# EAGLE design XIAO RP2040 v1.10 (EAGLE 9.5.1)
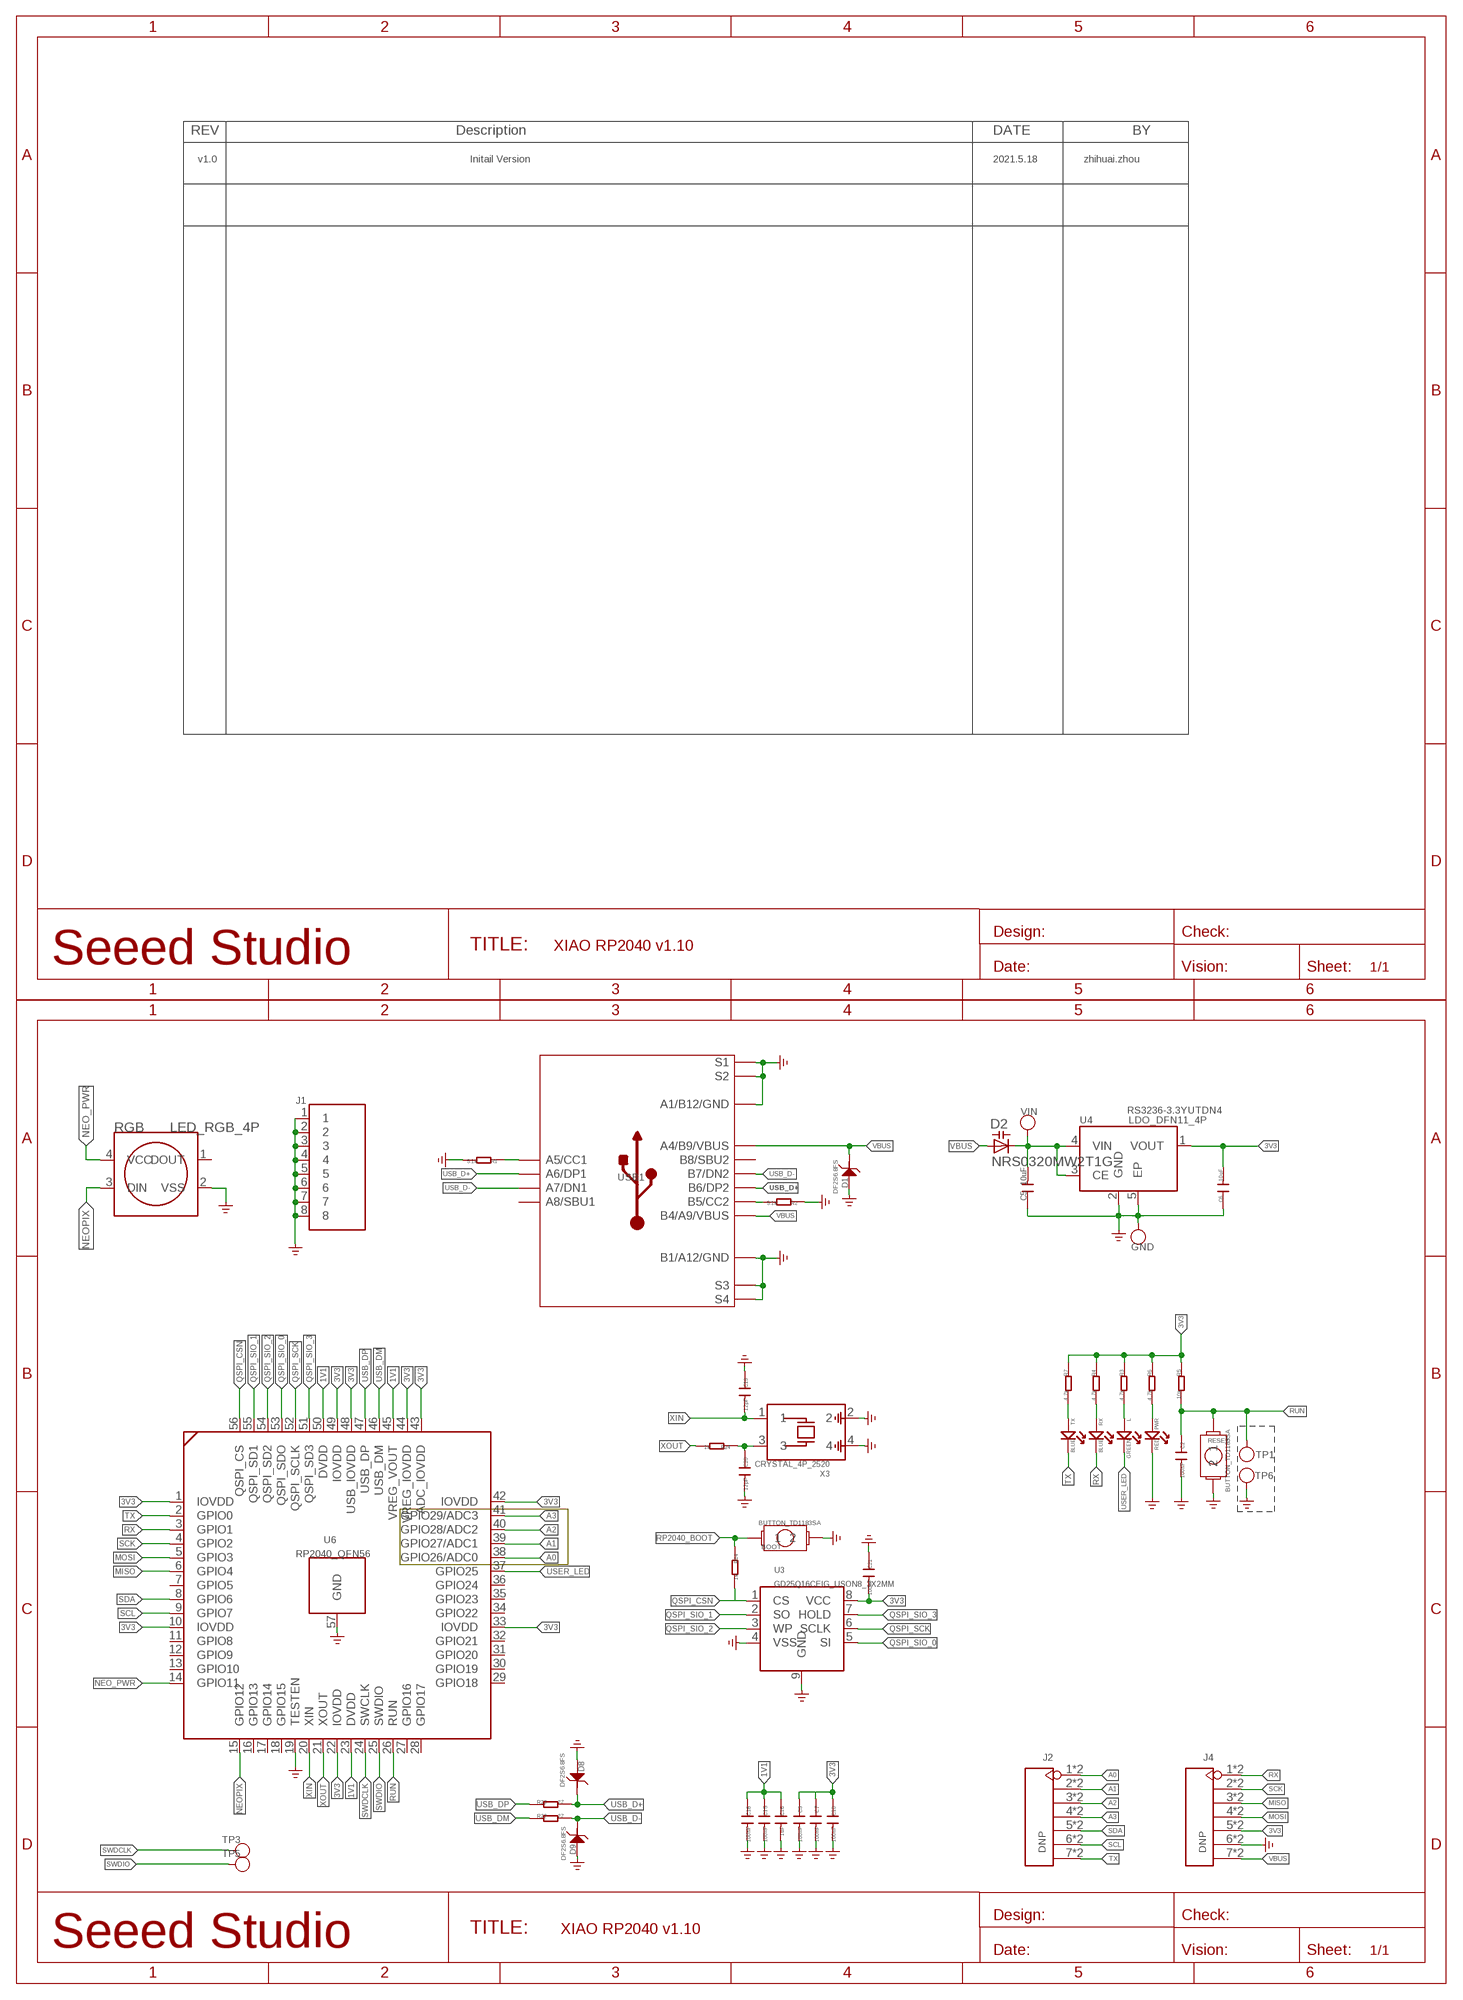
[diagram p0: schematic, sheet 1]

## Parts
BOOT  BUTTON_TD1183SA  [BUTTON_TD1183SA]
C2  100nF  CAP\0201NNS  [0201_NORMAL\NOSILK]
C3  100nF  CAP\0201NNS  [0201_NORMAL\NOSILK]
C5  10uF  C-0402  [C0402]
C6  10uF  C-0402  [C0402]
C7  100nF  CAP\0201NNS  [0201_NORMAL\NOSILK]
C10  100nF  CAP\0201NNS  [0201_NORMAL\NOSILK]
C15  100nF  CAP\0201NNS  [0201_NORMAL\NOSILK]
C16  1uF  CAP\0201NNS  [0201_NORMAL\NOSILK]
C18  100nF  CAP\0201NNS  [0201_NORMAL\NOSILK]
C19  12pF  CAP\0201NNS  [0201_NORMAL\NOSILK]
C20  12pF  CAP\0201NNS  [0201_NORMAL\NOSILK]
C21  100nF  CAP\0201NNS  [0201_NORMAL\NOSILK]
D1  DF2S6.8FS  D-ESD-2P'DF2S6.8FS'  [SOD-923]
D2  NRS0320MW2T1G  DIODE_CAPACITANCE-SOD523  [SOD523]
D8  DF2S6.8FS  D-ESD-2P'DF2S6.8FS'  [SOD-923]
D9  DF2S6.8FS  D-ESD-2P'DF2S6.8FS'  [SOD-923]
GND  TEST-POINT'4080'  [TP-80X40MIL]
J1  SHIELDING-COVER-XIAO_RP2040_PRD  [SHIELDING-COVER_XIAO_RP2040_PRD]
J2  DNP  HEADER-7P-HALF-HOLE-2.54  [H7-HALF-HOLE-2.54]
J4  DNP  HEADER-7P-HALF-HOLE-2.54  [H7-HALF-HOLE-2.54]
L  GREEN  LED-0402  [LED-0402]
PWR  RED  LED-0402  [LED-0402]
R1  5.1k  R-0201  [R0201]
R2  5.1k  R-0201  [R0201]
R3  4.7k  R-0201  [R0201]
R4  4.7k  R-0201  [R0201]
R5  10k  R-0201  [R0201]
R6  4.7k  R-0201  [R0201]
R7  4.7k  R-0201  [R0201]
R14  1k  R-0201  [R0201]
R22  27  R-0201  [R0201]
R23  27  R-0201  [R0201]
R24  1k  R-0201  [R0201]
RESET  BUTTON_TD1183SA  [BUTTON_TD1183SA]
RGB  LED_RGB_4P  [LED_RGB_2427]
RX  BLUE  LED-0402  [LED-0402]
TP1  TEST-POINT'4545'  [TP-D45MIL]
TP3  TEST-POINT'4545'  [TP-D45MIL]
TP5  TEST-POINT'4545'  [TP-D45MIL]
TP6  TEST-POINT'4545'  [TP-D45MIL]
TX  BLUE  LED-0402  [LED-0402]
U3  GD25Q16CEIG_USON8_3X2MM  [GD25Q16CEIG_USON8_3X2MM]
U4  LDO_DFN11_4P  [LDO_DFN1*1_4P]
U6  RP2040_QFN56  [RP2040_QFN56]
USB1  USB2.0-TYPE-C  [USB2.0-TYPE-C]
VIN  TEST-POINT'4080'  [TP-80X40MIL]
X3  CRYSTAL_4P_2520  [CRYSTAL_4P_2520]

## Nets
1V1: C15.1 C16.1 C18.1 U6.23(DVDD) U6.45(VREG_VOUT) U6.50(DVDD)
3V3: C3.1 C6.2 C7.1 C10.1 C21.2 J4.5 J4.17 R3.1 R4.1 R5.1 R6.1 R7.1 U3.8(VCC) U4.1(VOUT) U6.1(IOVDD) U6.10(IOVDD) U6.22(IOVDD) U6.33(IOVDD) U6.42(IOVDD) U6.43(ADC_IOVDD) U6.44(VREG_IOVDD) U6.48(USB_IOVDD) U6.49(IOVDD)
A0: J2.1 J2.13 U6.38(GPIO26/ADC0)
A1: J2.2 J2.14 U6.39(GPIO27/ADC1)
A2: J2.3 J2.15 U6.40(GPIO28/ADC2)
A3: J2.4 J2.16 U6.41(GPIO29/ADC3)
GND: BOOT.2 C2.2 C3.2 C5.1 C6.1 C7.2 C10.2 C15.2 C16.2 C18.2 C19.1 C20.2 C21.1 D1.2 D8.2 D9.2 GND.1(T) J1.1 J1.2 J1.3 J1.4 J1.5 J1.6 J1.7 J1.8 J4.6 J4.18 PWR.- R1.2 R2.1 RESET.2 RGB.2(VSS) TP6.T U3.4(VSS) U3.9(GND) U4.2(GND) U4.5(EP) U6.19(TESTEN) U6.57(GND) USB1.A1_B12(A1/B12/GND) USB1.B1_A12(B1/A12/GND) USB1.S1 USB1.S2 USB1.S3 USB1.S4 USB1.S5(S1) USB1.S6(S2) X3.2 X3.4 ; supply symbol labelled GND_POWER
MISO: J4.3 J4.15 U6.6(GPIO4)
MOSI: J4.4 J4.16 U6.5(GPIO3)
N$1: R1.1 USB1.A5(A5/CC1)
N$2: R2.2 USB1.B5(B5/CC2)
N$5: L.+ R3.2
N$6: R7.2 TX.+
N$8: C20.1 R24.1 X3.3
N$9: R4.2 RX.+
N$16: PWR.+ R6.2
NEO_PWR: RGB.4(VCC) U6.14(GPIO11)
NEOPIX: RGB.3(DIN) U6.15(GPIO12)
QSPI_CSN: R14.2 U3.1(CS) U6.56(QSPI_CS)
QSPI_SCK: U3.6(SCLK) U6.52(QSPI_SCLK)
QSPI_SIO_0: U3.5(SI) U6.53(QSPI_SDO)
QSPI_SIO_1: U3.2(SO) U6.55(QSPI_SD1)
QSPI_SIO_2: U3.3(WP) U6.54(QSPI_SD2)
QSPI_SIO_3: U3.7(HOLD) U6.51(QSPI_SD3)
RP2040_BOOT: BOOT.1 R14.1
RUN: C2.1 R5.2 RESET.1 TP1.T U6.26(RUN)
RX: J4.1 J4.13 RX.- U6.3(GPIO1)
SCK: J4.2 J4.14 U6.4(GPIO2)
SCL: J2.6 J2.18 U6.9(GPIO7)
SDA: J2.5 J2.17 U6.8(GPIO6)
SWDCLK: TP3.T U6.24(SWCLK)
SWDIO: TP5.T U6.25(SWDIO)
TX: J2.7 J2.19 TX.- U6.2(GPIO0)
USB_D+: D8.1 R23.2 USB1.A6(A6/DP1) USB1.B6(B6/DP2)
USB_D-: D9.1 R22.2 USB1.A7(A7/DN1) USB1.B7(B7/DN2)
USB_DM: R22.1 U6.46(USB_DM)
USB_DP: R23.1 U6.47(USB_DP)
USER_LED: L.- U6.37(GPIO25)
VBUS: D1.1 D2.A J4.7 J4.19 USB1.A4_B9(A4/B9/VBUS) USB1.B4_A9(B4/A9/VBUS)
VIN: C5.2 D2.C U4.3(CE) U4.4(VIN) VIN.1(T)
XIN: C19.2 U6.20(XIN) X3.1
XOUT: R24.2 U6.21(XOUT)
Unconnected: RGB.1(DOUT) U6.7(GPIO5) U6.11(GPIO8) U6.12(GPIO9) U6.13(GPIO10) U6.16(GPIO13) U6.17(GPIO14) U6.18(GPIO15) U6.27(GPIO16) U6.28(GPIO17) U6.29(GPIO18) U6.30(GPIO19) U6.31(GPIO20) U6.32(GPIO21) U6.34(GPIO22) U6.35(GPIO23) U6.36(GPIO24) USB1.A8(A8/SBU1) USB1.B8(B8/SBU2)

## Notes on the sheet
- v1.0 | Initail Version | 2021.5.18 | zhihuai.zhou
- RS3236-3.3YUTDN4

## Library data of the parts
BOOT RESET = BUTTON_TD1183SA:BUTTON_TD1183SA: 德艺隆:TD-1183SA/311020740
C2 C3 C7 C10 C15 C16 C18-C21 = Seeed-Discrete:CAP: Ceramic Capacitors
C5 C6 = XIAO RP2040 PRD v1.0:C*: Ceramic Capacitors
D1 D8 D9 = Discrete-new:D-ESD-2P: SOD-923:304060009;SOD-123:304060001
D2 = XIAO RP2040 PRD v1.0:DIODE_CAPACITANCE-: Capacity DIODE
GND VIN = Discrete-new:TEST-POINT
J1 = XIAO RP2040 PRD v1.0:SHIELDING-COVER-XIAO_RP2040_PRD
J2 J4 = Connector-new:HEADER-7P-HALF-HOLE
L PWR RX TX = Discrete-small:LED
R1-R7 R14 R22-R24 = XIAO RP2040 PRD v1.0:R*
RGB = XIAO RP2040 PRD v1.0:LED_RGB_4P
TP1 TP3 TP5 TP6 = Discrete-new:TEST-POINT; PARTNO: DNP
U3 = FLASH_GD25Q16CEIG_2:GD25Q16CEIG_USON8_3X2MM
U4 = LDO_DFN1X1_4P:LDO_DFN1*1_4P
U6 = RP2040_QFN56:RP2040_QFN56
USB1 = USB C:USB2.0-TYPE-C
X3 = CRYSTAL_4P:CRYSTAL_4P_2520

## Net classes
1 power: width 0.152 mm, drill 0.152 mm, clearance 0.152 mm
2 gnd: width 0.152 mm, drill 0.152 mm, clearance 0.152 mm
3 usbvcc: width 0.152 mm, drill 0.152 mm, clearance 0.152 mm

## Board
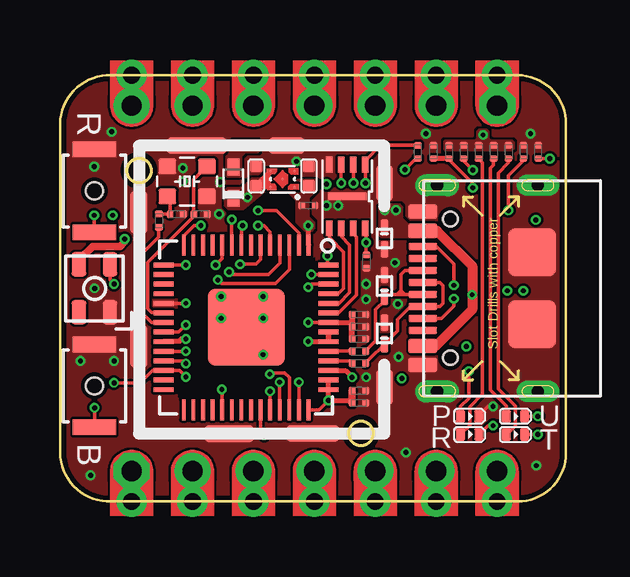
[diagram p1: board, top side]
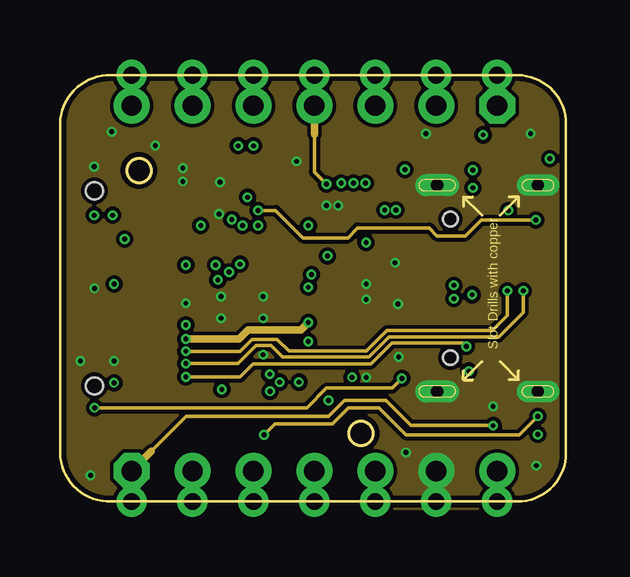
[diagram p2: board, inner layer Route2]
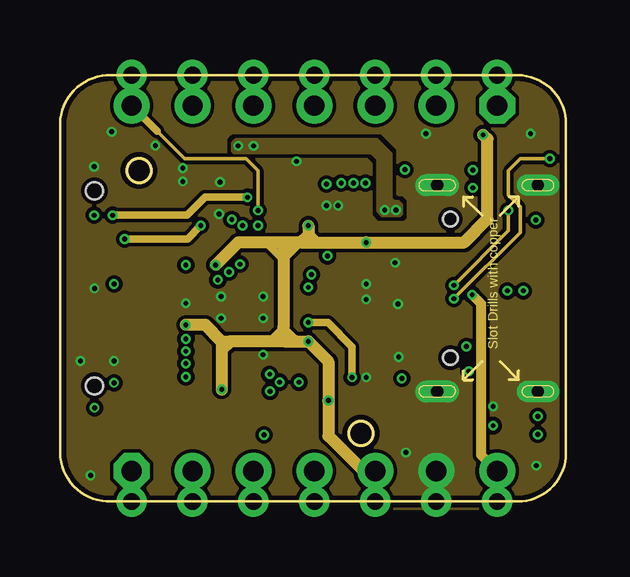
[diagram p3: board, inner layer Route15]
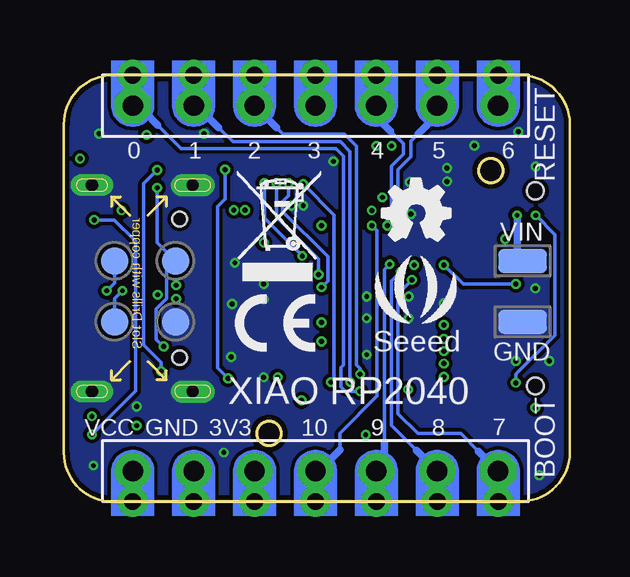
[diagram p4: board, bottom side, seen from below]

Size 21.1 x 17.78 mm. Coordinates in mm from the lower left corner, seen from the top.
Outline: 2.13,0 19.07,0 arc90 21.1,2.03 21.1,15.75 arc90 19.07,17.78 2.13,17.78 arc90 0,15.75 0,2.03 arc90 2.13,0
Copper layers (1+2*15+16): Top 0.035mm / dielectric 0.2mm / Route2 0.0175mm / dielectric 1.1mm / Route15 0.0175mm / dielectric 0.2mm / Bottom 0.035mm
Design rules "SeeedStudio_2layer_DRU_no_angle_20140221 *": minimum track width 1mil, minimum drill 8mil, track to track 4mil, track to pad 4mil, pad to pad 6mil, via to via 4mil, smd to smd 0mil, copper to edge 8mil, drill to drill 10mil, minimum pad ring 4mil, minimum via ring 4mil, stop-mask expansion 2mil, vias tented up to drill 25mil, thermal gap 0mil
tRestrict: area 4.9,4.3 to 10.6,10.2

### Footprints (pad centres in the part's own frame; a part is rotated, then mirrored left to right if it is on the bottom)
BUTTON_TD1183SA = smd 0.65 x 1.8: 1 -1.725,0; 2 1.725,0 | hole 0.7: 0,0
0201_NORMAL\NOSILK = smd 0.279 x 0.318: 1 -0.279,0; 2 0.279,0
C0402 = smd 0.508 x 0.508: 1 -0.406,0; 2 0.406,0
SOD-923 = smd 0.7 x 0.3: 1 -0.45,0; 2 0.45,0
SOD523 = smd 0.7 x 0.5: A 0.7,0; C -0.6,0
TP-80X40MIL = smd 2.032 x 1.016: 1 0,0
SHIELDING-COVER_XIAO_RP2040_PRD = smd 0.7 x 1.778: 1 -4.953,3.556; 2 -4.953,-2.032 | smd 2.032 x 0.7: 3 -1.18,-5.673 | smd 2.2 x 0.7: 4 2.29,-5.668 | smd 0.7 x 1.5: 5 5.283,-3.737; 6 5.283,4.772 | smd 1.5 x 0.7: 7 1.216,6.332 | smd 2.5 x 0.7: 8 -2.54,6.332 | hole 1: -4.953,5.3; 4.3,-5.672
H7-HALF-HOLE-2.54 = drill 0.85 pad 1.5 octagon: 1 0,7.62 | drill 0.85 pad 1.5: 2 0,5.08; 3 0,2.54; 4 0,0; 5 0,-2.54; 6 0,-5.08; 7 0,-7.62 | drill 0.7 pad 1.27: 13 -1.27,7.62; 14 -1.27,5.08; 15 -1.27,2.54; 16 -1.27,0; 17 -1.27,-2.54; 18 -1.27,-5.08; 19 -1.27,-7.62
LED-0402 = smd 0.385 x 0.508: + -0.383,0; - 0.383,0
R0201 = smd 0.279 x 0.318: 1 -0.279,0; 2 0.279,0
LED_RGB_2427 = smd 1 x 0.6: 1 1,-0.65; 2 1,0.65; 3 -1,0.65; 4 -1,-0.65
TP-D45MIL = smd 1.143 x 1.143: T 0,0
GD25Q16CEIG_USON8_3X2MM = smd 0.65 x 0.3: 1 -1.33,0.75; 2 -1.33,0.25; 3 -1.33,-0.25; 4 -1.33,-0.75; 5 1.33,-0.75; 6 1.33,-0.25; 7 1.33,0.25; 8 1.33,0.75 | smd 0.3 x 1.6: 9 0,0
LDO_DFN1*1_4P = smd 0.1 x 0.1: 1 -0.33,-0.5; 2 0.33,-0.5; 3 0.33,0.51; 4 -0.33,0.5; 5 0,0
RP2040_QFN56 = smd 0.875 x 0.2: 1 -3.438,2.6; 2 -3.438,2.2; 3 -3.438,1.8; 4 -3.438,1.4; 5 -3.438,1; 6 -3.438,0.6; 7 -3.438,0.2; 8 -3.438,-0.2; 9 -3.438,-0.6; 10 -3.438,-1; 11 -3.438,-1.4; 12 -3.438,-1.8; 13 -3.438,-2.2; 14 -3.438,-2.6; 29 3.438,-2.6; 30 3.438,-2.2; 31 3.438,-1.8; 32 3.438,-1.4; 33 3.438,-1; 34 3.438,-0.6; 35 3.438,-0.2; 36 3.438,0.2; 37 3.438,0.6; 38 3.438,1; 39 3.438,1.4; 40 3.438,1.8; 41 3.438,2.2; 42 3.438,2.6 | smd 0.2 x 0.875: 15 -2.6,-3.438; 16 -2.2,-3.438; 17 -1.8,-3.438; 18 -1.4,-3.438; 19 -1,-3.438; 20 -0.6,-3.438; 21 -0.2,-3.438; 22 0.2,-3.438; 23 0.6,-3.438; 24 1,-3.438; 25 1.4,-3.438; 26 1.8,-3.438; 27 2.2,-3.438; 28 2.6,-3.438; 43 2.6,3.438; 44 2.2,3.438; 45 1.8,3.438; 46 1.4,3.438; 47 1,3.438; 48 0.6,3.438; 49 0.2,3.438; 50 -0.2,3.438; 51 -0.6,3.438; 52 -1,3.438; 53 -1.4,3.438; 54 -1.8,3.438; 55 -2.2,3.438; 56 -2.6,3.438 | smd 3.2 x 3.2: 57 0,0
USB2.0-TYPE-C = smd 1.2 x 0.6: A1_B12 0.05,3.2; A4_B9 0.05,2.4; B1_A12 0.05,-3.2; B4_A9 0.05,-2.4 | smd 1.2 x 0.3: A5 0.05,1.25; A6 0.05,0.25; A7 0.05,-0.25; A8 0.05,-1.25; B5 0.05,-1.75; B6 0.05,-0.75; B7 0.05,0.75; B8 0.05,1.75 | drill 0.508 pad 0.889 long: S1 -4.75,4.3; S2 -4.75,-4.3 | drill 0.508 pad 0.914 long: S3 -0.55,4.3; S4 -0.55,-4.3 | smd 2 x 2: S5 -4.5,1.5; S6 -4.5,-1.5 | hole 0.6: -1.1,-2.89; -1.1,2.89
CRYSTAL_4P_2520 = smd 0.75 x 0.65: 1 -0.825,-0.625; 2 0.825,-0.625; 3 0.825,0.625; 4 -0.825,0.625

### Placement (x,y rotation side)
BOOT  1.44,4.83 90 top
C2  15.57,14.58 90 top
C3  10.36,12.34 0 top
C5  8.18,13.58 270 top
C6  10.38,13.58 270 top
C7  12.46,4.62 0 top
C10  12.46,4.11 0 top
C15  12.46,7.8 0 top
C16  12.46,6.78 0 top
C18  12.46,7.29 0 top
C19  5.87,11.97 180 top
C20  4.87,11.97 0 top
C21  12.78,10.01 90 top
D1  13.53,10.97 270 top
D2  7.23,13.25 90 top
D8  13.53,8.99 90 top
D9  13.53,7.01 90 top
GND  1.97,7.49 0 bottom
J1  8.25,8.51 0 top
J2  10.61,16.51 270 top
J4  10.61,1.27 90 top
L  18.99,3.56 0 top
PWR  17.09,3.56 0 top
R1  19.94,14.58 90 top
R2  19.32,14.58 270 top
R3  18.08,14.58 270 top
R4  17.46,14.58 270 top
R5  16.22,14.58 270 top
R6  16.84,14.58 270 top
R7  18.7,14.58 270 top
R14  14.93,14.58 90 top
R22  12.46,5.77 0 top
R23  12.46,6.27 0 top
R24  4.12,11.71 270 top
RESET  1.44,12.95 90 top
RGB  1.44,8.89 270 top
RX  17.09,2.79 0 top
TP1  16.45,10.03 0 bottom
TP3  18.99,7.49 0 bottom
TP5  18.99,10.03 0 bottom
TP6  16.45,7.49 0 bottom
TX  18.99,2.79 0 top
U3  11.98,12.73 270 top
U4  9.29,13.44 90 top
U6  7.76,7.26 270 top
U$4  [OSHW_FILLX100_NOTEXT]  7.82,10.9 0 bottom
U$6  [SEEED-SILK--TNAME-160*153MIL]  6.4,8.93 0 bottom
USB1  15.18,8.89 180 top
VIN  1.97,10.03 180 bottom
X3  5.3,13.35 180 top

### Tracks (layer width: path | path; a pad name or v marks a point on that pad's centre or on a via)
1V1  (via drill 0.2 pad 0.41)
  Top 0.152: v10.36,7.46 U6.50
  Top 0.203: U6.50 12.18,7.46 C18.1 | U6.23 4.34,6.68 4.97,6.68 5.07,6.78 v5.25,6.78 | U6.45 11.9,5.46 v12.18,5.18
  Top 0.254: C15.1 C18.1 C16.1
  Route2 0.305: v5.25,6.78 7.48,6.78 7.85,7.16 10.05,7.16 v10.36,7.46
  Route15 0.305: v12.18,5.18 12.18,6.45 11.17,7.46 v10.36,7.46
3V3  (via drill 0.2 pad 0.41)
  Top 0.152: U6.22 4.95,7.06 v5.25,7.37 | v11.19,4.22 10.8,3.83 U6.42 | U3.8 12.77,11.36 v12.77,10.8 12.77,10.3 C21.2 | v6.75,4.67 6.76,4.66 U6.33 | v6.49,9.87 6.76,10.14 U6.10
  Top 0.203: U6.48 U6.49 11.2,6.68 v10.36,6.68 | U6.44 U6.43 v11.19,4.22 12.08,4.22 C10.1 | U6.42 10.38,3.84 | U6.1 v10.36,11.51
  Top 0.254: J4.5 J4.17
  Top 0.305: C10.1 C7.1
  Route15 0.305: 8.59,10.8 9.26,10.14 9.31,10.14 9.37,10.14 10.04,10.8 | 8.59,6.68 8.73,6.68 9.31,7.26 9.85,6.73 9.85,6.68
  Route15 0.508: 9.34,6.68 9.85,6.68 v10.36,6.68 11.19,5.84 v11.19,4.22 11.19,2.73 12.66,1.27 J4.5 | 9.34,6.68 8.59,6.68 7.1,6.68 | 6.75,6.68 7.1,6.68 | 10.36,10.8 10.67,10.8 | v10.36,11.51 10.36,11.12 | 10.36,11.12 10.36,10.8 | 10.04,10.8 10.36,10.8 | 10.04,10.8 9.31,10.8 | 9.31,10.8 8.59,10.8 7.43,10.8 v6.49,9.87 | 7.1,6.68 6.75,6.33 | 10.04,10.8 10.36,11.12 | 10.36,11.12 10.67,10.8 | 9.31,10.8 9.31,10.14 9.31,7.26 9.31,6.71 9.34,6.68 | 6.75,6.68 6.75,6.33 | v17.65,15.29 17.82,15.11 17.82,11.77 16.85,10.8 v12.77,10.8 10.67,10.8 | v5.25,7.37 6.06,7.37 6.75,6.68 | 6.75,6.33 v6.75,4.67
  pour Top: 9.5,13.06 9.9,13.45 10.63,13.45 10.72,13.36 10.72,12.99 10.38,12.65 10.38,11.89 10.62,11.65 10.62,11.38 10.51,11.26 10.22,11.26 9.85,11.63 9.85,12.55 9.5,12.89
  pour Top: 16.06,15.07 15.99,15.01 15.99,14.69 16.06,14.63 18.85,14.63 18.97,14.74 18.97,14.96 18.86,15.06 17.99,15.06 17.91,15.14 17.91,15.43 17.81,15.53 17.47,15.53 17.37,15.43 17.37,15.14 17.3,15.07
A0  (via drill 0.2 pad 0.41)
  Top 0.152: v8.76,4.6 U6.38
  Top 0.254: J2.1 J2.13
  Bottom 0.152: 17.19,15.7 16.21,14.72 9.75,14.72 9.44,14.41 9.44,5.7 9.54,5.6 9.54,4.79 9.35,4.6 9,4.6 v8.76,4.6
  Bottom 0.305: 17.19,15.7 17.72,16.23 17.95,16.23 J2.1
A1  (via drill 0.2 pad 0.41)
  Top 0.152: v9.16,4.98 U6.39
  Top 0.254: J2.2 J2.14
  Bottom 0.102: J2.2 15.69,16
  Bottom 0.152: 14.65,15.6 14.05,15 9.57,15 9.16,14.59 v9.16,4.98
  Bottom 0.305: 14.65,15.6 15.08,16.03 15.66,16.03 15.69,16
A2  (via drill 0.2 pad 0.41)
  Top 0.152: U6.40 9.57,5.17 9.36,5.37 8.81,5.37 v8.75,5.31
  Top 0.254: J2.3 J2.15
  Bottom 0.152: 12.34,15.7 12.34,15.65 | v8.75,5.31 8.75,5.55 8.9,5.7 8.9,14.82 9.39,15.32 11.96,15.32 12.24,15.6
  Bottom 0.305: J2.3 12.34,15.7 12.24,15.6
A3  (via drill 0.2 pad 0.41)
  Top 0.152: v9.96,4.98 U6.41
  Top 0.254: J2.4 J2.16
  Route2 0.152: 10.61,15.32 10.61,13.74 v11.12,13.23
  Route2 0.305: J2.4 10.61,15.32
  Bottom 0.152: v9.96,4.98 9.83,5.11 9.83,11.95 v11.12,13.23
GND  (via drill 0.2 pad 0.41)
  Top 0.152: v18.06,3.96 17.84,3.96 17.47,3.59 PWR.- | v5.25,8.27 v5.25,8.26 U6.19
  Top 0.305: U6.57 7.76,6.83 v8.48,6.12
  other vias: 8.48,7.65 6.72,7.65 8.48,8.55 1.44,8.89 0.86,5.87 2.25,5.87 1.43,13.97 2.15,15.42 3.98,14.85 6.68,13.32 11.12,12.34 11.6,12.34 12.77,8.43 12.77,9.07 12.77,5.18 1.28,1.09 19.87,1.5 14.43,2.04 19.63,15.34 15.26,15.34 6.72,8.55 5.12,13.91 9.86,14.19 14.13,6.03 14.09,8.24 13.98,9.96 6.63,11.99 5.12,13.35
  pour Top (rank 3, no thermals): -0.19,17.93 21.51,17.93 21.53,17.91 21.53,-0.28 3.88,-0.28 3.88,-0.91 2.08,-0.91 2.08,-0.25 -0.21,-0.25
  pour Route2 (isolate 0.152, rank 6, no thermals): -0.19,17.93 21.51,17.93 21.53,17.91 21.53,-0.28 3.88,-0.28 3.85,-1.24 2.08,-1.24 2.08,-0.25 -0.21,-0.25
  pour Route15 (isolate 0.152, rank 6, no thermals): -0.19,17.93 21.51,17.93 21.53,17.91 21.53,-0.28 3.88,-0.28 3.85,-1.57 2.08,-1.57 2.08,-0.25 -0.21,-0.25
  pour Bottom (isolate 0.152, rank 6, no thermals): -0.19,17.93 21.51,17.93 21.53,17.91 21.53,-0.28 3.88,-0.28 3.85,-1.93 2.08,-1.93 2.08,-0.25 -0.21,-0.25
MISO  (via drill 0.2 pad 0.41)
  Top 0.152: U6.6 8.37,10.69 8.37,10.08 8.19,9.9 v7.51,9.9
  Top 0.254: J4.3 J4.15
  Bottom 0.152: v7.51,9.9 7.74,9.67 7.74,2.49
  Bottom 0.305: J4.3 7.74,1.6 7.74,2.49
MOSI  (via drill 0.2 pad 0.41)
  Top 0.152: U6.5 8.76,11.24 8.5,11.51 v8.26,11.51
  Top 0.254: J4.4 J4.16
  Bottom 0.152: 9.59,2.15 9.59,2.85 8.04,4.39 8.04,11.29 v8.26,11.51
  Bottom 0.305: 9.59,2.15 10.47,1.27 J4.4
N$1  (via drill 0.2 pad 0.41)
  Top 0.152: USB1.A5 15.91,7.64 16.43,8.15 v16.43,8.46 | R1.1 v20.43,14.3
  Route15 0.152: v16.43,8.46 19.19,11.23 19.19,12.29 18.7,12.79 18.7,13.79 19.21,14.3 v20.43,14.3
N$2  (via drill 0.2 pad 0.41)
  Top 0.152: USB1.B5 15.69,10.64 16.43,9.91 v16.43,9.02 | v18.7,12.14 18.7,13.59 19.32,14.21 R2.2
  Route15 0.152: v16.43,9.02 18.7,11.29 v18.7,12.14
N$5
  Top 0.152: R3.2 18.08,14.04 17.95,13.91 17.95,4.65 18.61,3.99 L.+
N$6
  Top 0.152: TX.+ 18.64,2.79 18.99,3.15 18.99,3.99 18.28,4.7 18.28,13.7 18.7,14.12 R7.2
N$8
  Top 0.152: R24.1 4.57,11.99 C20.1 4.59,12.61 X3.3
N$9
  Top 0.152: RX.+ 17.09,3.18 17.09,3.95 17.62,4.48 17.62,14.14 R4.2
N$16  (via drill 0.2 pad 0.41)
  Top 0.152: PWR.+ 16.7,3.96 17.05,4.31 v17.05,5.44 | R6.2 16.84,14.2 v17.21,13.82
  Bottom 0.152: v17.21,13.82 17.77,13.26 17.77,6.53 17.05,5.8 v17.05,5.44
NEO_PWR  (via drill 0.2 pad 0.41)
  Top 0.152: RGB.4 0.79,10.07 | U6.14 5.16,11.08 5.59,11.51 v5.87,11.51
  Top 0.305: 0.79,10.07 1.37,10.64 2.5,10.64 2.7,10.84 v2.7,10.95
  Route15 0.305: v2.7,10.95 5.31,10.95 v5.87,11.51
NEOPIX  (via drill 0.2 pad 0.41)
  Top 0.152: v5.25,9.87 U6.15 | 2.09,9.49 RGB.3 2.09,9.23 v2.25,9.07
  Bottom 0.152: v2.25,9.07 4.45,9.07 v5.25,9.87
QSPI_CSN  (via drill 0.2 pad 0.41)
  Top 0.152: v11.16,10.25 11.15,10.24 11.15,9.92 U6.56 | R14.2 13.37,14.86 12.73,14.22 U3.1 12.74,14.04 v12.74,13.28
  Bottom 0.152: v11.16,10.25 12.74,11.83 v12.74,13.28
QSPI_SCK
  Top 0.152: U3.6 11.73,11.05 12.08,10.7 12.08,8.72 11.63,8.26 U6.52
QSPI_SIO_0
  Top 0.152: 11.28,11.23 11.28,11.35 U3.5 11.23,11.01 11.83,10.41 11.83,8.89 11.6,8.66 U6.53
QSPI_SIO_1  (via drill 0.2 pad 0.41)
  Top 0.152: v10.48,9.47 v10.49,9.46 U6.55 | v12.24,13.28 U3.2
  Bottom 0.152: 12.24,13.31 v12.24,13.28 12.24,11.86 10.48,10.11 v10.48,9.47
QSPI_SIO_2  (via drill 0.2 pad 0.41)
  Top 0.152: v11.73,13.28 U3.3 | v10.36,8.94 10.48,9.06 U6.54
  Bottom 0.152: v11.73,13.28 11.73,12.76 11.98,12.5 11.98,12.09 10.1,10.21 10.1,9.2 v10.36,8.94
QSPI_SIO_3
  Top 0.152: U6.51 11.61,7.86 12.37,8.62 12.37,11.04 12.23,11.18 U3.7
RP2040_BOOT  (via drill 0.2 pad 0.41)
  Top 0.152: v1.44,3.91 BOOT.1 | R14.1 14.84,14.3 v14.38,13.84
  Route2 0.152: v1.44,3.91 10.29,3.91 11.12,4.74 13.86,4.74 v14.25,5.13
  Bottom 0.152: v14.25,5.13 14.7,5.58 14.7,12.29 14.38,12.61 v14.38,13.84
RUN  (via drill 0.2 pad 0.41)
  Top 0.152: RESET.1 1.43,11.24 v1.43,11.94 | v17.21,13.08 17.21,13.27 16.22,14.27 R5.2 | v2.25,4.95 3.35,4.95 3.86,5.46 U6.26 4.98,5.46 v5.25,5.19
  Top 0.203: R5.2 C2.1
  Route2 0.152: v16.95,6.46 16.81,6.6 13.84,6.6 12.97,5.74 8.06,5.74 7.51,5.19 v5.25,5.19
  Bottom 0.152: v17.21,13.08 17.21,10.79 TP1.T 16.81,9.68 16.81,8.46 17.25,8.02 17.25,6.77 v16.95,6.46 | v1.43,11.94 0.63,11.14 0.63,6.93 2.16,5.4 2.24,5.32 2.25,5.31 v2.25,4.95
RX  (via drill 0.2 pad 0.41)
  Top 0.152: v6.58,9.25 6.74,9.09 8.98,9.09 9.57,9.68 U6.3 | J4.1 2.99,0.33 | RX.- 17.84,3.16 v18.06,3.16 v18.06,3.17
  Top 0.254: J4.1 J4.13
  Route2 0.152: v18.06,3.17 14.64,3.17 13.59,4.22 11.87,4.22 11.19,3.54 5.26,3.54 3.8,2.08
  Route2 0.305: J4.1 3.8,2.08
  Bottom 0.152: 3.81,2.09 4.55,2.83 6.34,2.83 7.17,3.66 7.17,8.66 v6.58,9.25 | v6.58,9.25
  Bottom 0.305: J4.1 3.81,2.09
SCK  (via drill 0.2 pad 0.41)
  Top 0.152: v7.06,9.57 7.16,9.47 8.7,9.47 9.17,9.94 9.17,10.69 U6.4
  Top 0.254: J4.2 J4.14
  Bottom 0.152: 6.4,2.14 7.43,3.18 7.43,9.2 v7.06,9.57
  Bottom 0.305: J4.2 6.4,2.14
SCL  (via drill 0.2 pad 0.41)
  Top 0.152: U6.9 v7.16,11.76 v7.17,11.76
  Top 0.254: J2.6 J2.18
  Bottom 0.152: v7.17,11.76 7.17,13.84 6.63,14.38 6.63,15.02 6.33,15.33
  Bottom 0.305: J2.6 5.53,16.13 6.33,15.33
SDA  (via drill 0.2 pad 0.41)
  Top 0.152: U6.8 7.56,11.46 v7.61,11.51
  Top 0.254: J2.5 J2.17
  Bottom 0.152: v7.61,11.51 7.61,11.87 7.43,12.05 7.43,14 6.95,14.48 6.95,14.92 7.49,15.46
  Bottom 0.305: J2.5 8.07,16.04 7.49,15.46
SWDCLK  (via drill 0.2 pad 0.41)
  Top 0.152: v5.25,6.27 U6.24
  Route2 0.152: v5.25,6.27 7.52,6.27 8.01,6.76 9.05,6.76 9.54,6.27 10.14,6.27 12.78,6.27 13.63,7.13 18.03,7.13 18.66,7.76 v18.66,8.79
  Bottom 0.152: v18.66,8.79 18.99,8.46 TP3.T
SWDIO  (via drill 0.2 pad 0.41)
  Top 0.152: v5.25,5.75 5.14,5.86 U6.25
  Route2 0.152: v5.25,5.75 7.43,5.75 8.17,6.5 8.79,6.5 9.28,6.02 12.88,6.02 13.72,6.86 18.29,6.86 19.32,7.89 v19.32,8.79
  Bottom 0.152: v19.32,8.79 18.99,9.12 TP5.T
TX  (via drill 0.2 pad 0.41)
  Top 0.152: U6.2 9.96,11.2 9.02,12.14 v8.26,12.14 | TX.- v19.93,2.79
  Top 0.254: J2.7 J2.19
  Route2 0.152: v8.26,12.14 9,12.14 10.14,11 12.01,11 12.41,11.41 15.4,11.41 15.73,11.07 16.91,11.07 17.58,11.75 v19.84,11.75
  Route15 0.152: v8.26,12.14 8.26,13.8 7.76,14.3 5.2,14.3 4.06,15.44
  Route15 0.305: 4.06,15.44 J2.7
  Bottom 0.152: v19.84,11.75 19,11.75 18.12,10.86 18.12,4.61 v19.93,2.79
USB_D+
  Top 0.102: USB1.A6
  Top 0.152: USB1.B6 14.38,9.64 14.22,9.47 14.22,8.8 | R23.2 12.91,6.45 12.92,6.45 13.16,6.69 13.16,8 13.53,8.37 D8.1 13.62,8.54 13.72,8.64 | 13.63,8.64 13.72,8.64 | 13.72,8.64 13.92,8.64 14.05,8.64 | 14.05,8.64 14.22,8.64 | 14.22,8.64 14.38,8.64 | 14.38,8.64 USB1.A6 | 14.22,8.8 14.22,8.64 | 14.05,8.64 14.22,8.8 | 14.22,8.8 14.38,8.64
USB_D-
  Top 0.152: USB1.A7 15.84,9.14 15.97,9.02 15.97,8.26 15.85,8.14 USB1.B7 15.12,8.13 14.62,8.13 14.08,7.59 14.08,7.11 D9.1 12.92,5.94 12.91,5.94 R22.2
USB_DM
  Top 0.152: U6.46 12.09,5.86 R22.1
USB_DP
  Top 0.152: R23.1 11.2,6.27 U6.47
USER_LED  (via drill 0.2 pad 0.41)
  Top 0.152: v19.93,3.56 L.- | U6.37 8.36,2.93 v8.51,2.78
  Route2 0.152: v8.51,2.78 8.97,3.24 11.37,3.24 12.03,3.9 13.31,3.9 14.42,2.78 19.16,2.78 v19.93,3.56
VBUS  (via drill 0.2 pad 0.41)
  Top 0.254: J4.7 J4.19
  Top 0.406: USB1.B4_A9 15.73,11.29 17.19,9.83 v17.19,8.62 17.19,8 15.69,6.5 15.14,6.5 USB1.A4_B9
  Route15 0.406: v17.19,8.62 17.56,8.26 17.56,1.94 J4.7
  other vias: 13.54,12.15 14.01,12.15 7.43,14.83 8.07,14.83
  pour Bottom (isolate 0.254, no thermals): 18.38,1.37 18,0.99 17.72,0.99
  pour Top: 13.38,11.01 15.64,11.01 15.69,11.06 15.69,11.53 15.65,11.57 14.53,11.57 14.31,11.8 14.31,12.08 14.31,12.28 14.18,12.41 13.42,12.41 13.28,12.27 13.28,11.98 13.28,11.11
  pour Top: 6.96,13.54 7.54,13.54 7.59,13.59 7.59,14.4 7.74,14.55 8.26,14.55 8.35,14.64 8.35,14.97 8.25,15.07 7.23,15.07 6.9,14.74 6.9,13.6
  pour Route15: 7.27,15.09 7.13,14.95 7.13,14.62 7.24,14.5 7.5,14.5 12.97,14.5 13.19,14.29 13.19,12.1 13.4,11.89 14.2,11.89 14.31,11.99 14.31,12.38 14.14,12.55 13.96,12.55 13.87,12.64 13.87,14.5 13.4,14.97 13.24,15.14 7.4,15.14 7.32,15.14
VIN  (via drill 0.2 pad 0.41)
  Top 0.152: C5.2 8.21,13.2 | C5.2 8.43,13.41 8.49,13.41 | 8.62,13.29 8.49,13.41 | 8.62,13.6 8.62,13.29 | U4.4 8.24,13.11 C5.2 | C5.2 8.35,13.17 | 8.35,13.17 8.5,13.17 8.62,13.29 | 8.49,13.41 8.49,13.31 8.35,13.17 | U4.3 8.7,13.69 8.7,13.2
  Top 0.254: U4.4 8.7,13.2 8.49,13.41 | U4.3 C5.2
  Route15 0.305: v2.2,11.94 5.3,11.94 6.05,12.69 v7.82,12.69
  Bottom 0.305: 2.3,9.98 2.28,10.01 1.52,10.01 | VIN.1 2.2,10.26 v2.2,11.94
  Bottom 0.406: VIN.1 1.31,10.03 1.34,10.01 1.52,10.01
  pour Top: 7.99,13.49 7.6,13.09 6.96,13.09 6.84,12.97 6.84,12.34 7.02,12.17 7.66,12.17 8.75,13.1 8.36,13.49
XIN
  Top 0.152: U6.20 4.32,7.87 3.83,7.87 3.65,8.05 3.65,9.97 5.59,11.9 C19.2 5.58,11.99 5.58,13.42 X3.1
XOUT
  Top 0.152: U6.21 3.83,7.46 3.35,7.95 3.35,10.26 4.12,11.04 R24.2

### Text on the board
tPlace: R | B
tNames: P | U | R | T
bNames: 6 | 5 | 4 | 3 | 2 | 1 | 0 | VIN | GND | Seeed | XIAO RP2040 | 7 | 8 | 9 | 10 | 3V3 | GND | VCC
tTest: RUN | BOOT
